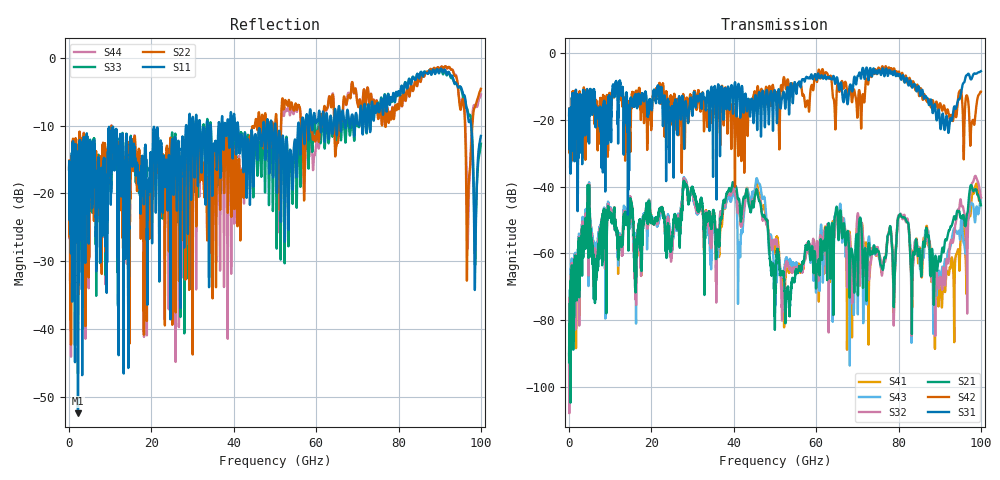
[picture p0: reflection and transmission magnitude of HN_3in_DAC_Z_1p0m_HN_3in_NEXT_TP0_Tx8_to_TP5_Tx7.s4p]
# GHz S RI R 45
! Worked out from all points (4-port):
!   4000 points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, 25 MHz to 100 GHz, reference 45 ohm
!   strongest paths, dB at 25 MHz, 25.02 GHz, 50.02 GHz, 75.03 GHz, 100 GHz:
!     S31: -18.6, -16.5, -11.2, -5.4, -5.4
!     S42: -18.6, -16.6, -12.4, -4.6, -11.5
!     S21: -90.2, -55.2, -72.8, -59.5, -45.6
!     S32: -92.3, -57.4, -57.3, -58.8, -43.4
!     S43: -88.3, -57.0, -74.5, -59.9, -43.5
!     S41: -89.5, -55.8, -58.1, -59.3, -43.4
!   lowest |S11| = -52.5 dB at 2.175 GHz (marker M1), VSWR 1.00, Z = 44.8 + j0.0812 ohm
!   |S11| at or under -10 dB: start of sweep to 28.4 GHz; 41.04 GHz to 47.14 GHz (6.101 GHz wide, 13.8 % of centre); 50.13 GHz to 55.61 GHz (5.475 GHz wide, 10.4 % of centre)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
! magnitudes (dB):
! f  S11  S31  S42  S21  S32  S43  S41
! 25 MHz  -16.4  -18.6  -18.6  -90.2  -92.3  -88.3  -89.5
! 2.175 GHz  -52.5  -28.5  -26.7  -66.2  -63.9  -60.9  -63.6
! 45.67 GHz  -15.0  -22.7  -10.7  -41.2  -40.9  -37.7  -39.3
! 53 GHz  -13.9  -10.2  -8.1  -71.0  -62.9  -62.2  -63.6
! 80.4 GHz  -5.5  -6.7  -7.2  -48.3  -48.4  -48.2  -48.4
! 90.1 GHz  -1.7  -21.6  -15.0  -62.4  -67.1  -67.7  -68.1
! 100 GHz  -11.5  -5.4  -11.5  -45.6  -43.4  -43.5  -43.4
